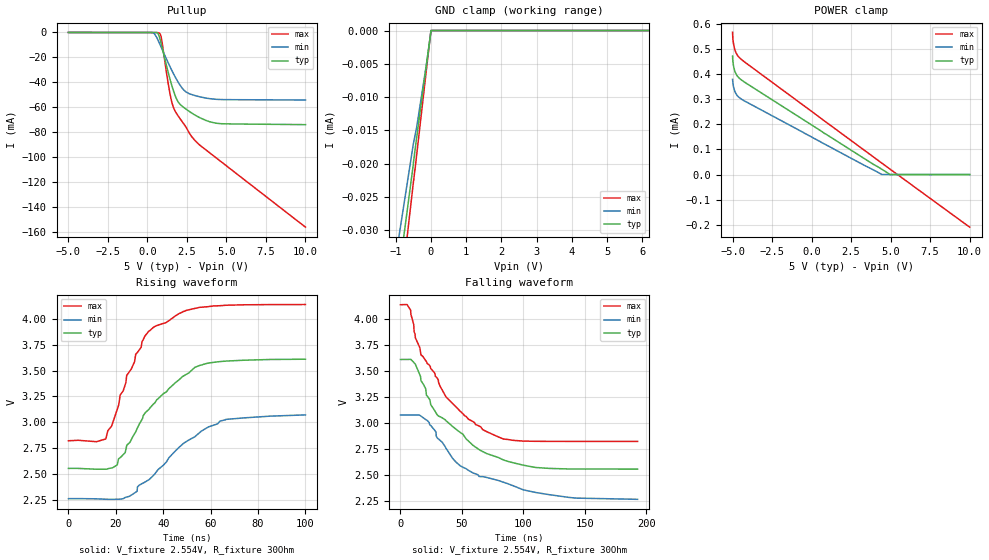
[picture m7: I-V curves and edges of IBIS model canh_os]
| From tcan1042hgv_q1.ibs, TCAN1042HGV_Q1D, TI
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|   canh_os Model
[Model]   canh_os
Model_type   I/O_open_source
Polarity   Inverting
Enable   Active-Low
Vinl = 0.5
Vinh = 0.9
Vmeas = 3
Vref = 2.554
Cref = 2pF
Rref = 30
|   typ   min   max
|   (nom PVT)   (fast PVT)   (slow PVT)
C_comp   8.777e-12   8.206e-12   9.702e-12
| Where nom  PVT is Nominal Process, 5V, 27C
|   Fast PVT is Strong Process,  5.5V, -55C
|   Slow PVT is Weak Process,   4.5V, 150C
[Voltage Range]   5   4.5   5.5
|Junction Temperature
[Temperature Range]   27   150   -55
[Pullup Reference]   5   4.5   5.5
[Pulldown Reference]   0   0   0
[Power Clamp Reference]   5   4.5   5.5
[GND Clamp Reference]   0   0   0
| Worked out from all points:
|   slope of the pullup table from 0 to 0.75 V, typ, clamps not added: 231 ohm
|   falling waveform, V_fixture 2.554V, R_fixture 30Ohm: 20-80 % time 44.1ns typ, 55.6ns min, 39.9ns max; typ from 3.61 V to 2.55 V
|   rising waveform, V_fixture 2.554V, R_fixture 30Ohm: 20-80 % time 21.5ns typ, 23.4ns min, 13.7ns max; typ from 2.55 V to 3.61 V
[GND Clamp]
|   Voltage   I(typ)   I(min)   I(max)
-5V       -202.4uA   -171.2uA   -233.7uA
-3.357V   -134.6uA   -114.5uA   -155.4uA
-500mV    -20.15uA   -17.09uA   -22.94uA
-495.5mV  -19.75uA   -16.97uA   -22.73uA
-455mV    -18.15uA   -15.9uA    -20.94uA
-450.5mV  -17.97uA   -15.78uA   -20.93uA
-405.5mV  -16.14uA   -14.59uA   -18.77uA
-108.5mV  -4.381uA   -4.46uA    -5.008uA
-5mV      -411.1nA   -364.3nA   -280.6nA
-500uV    -238.5nA   0A         0A
45mV      0A         0A         0A
10V       0A         0A         0A
[Pullup]
|   Voltage   I(typ)   I(min)   I(max)
-5V       -31.53uA   57.79uA    -113.1uA
296.5mV   -97.64uA   -126.2uA   -124.8uA
632mV     -357.2uA   -5.205mA   -176.4uA
760mV     -3.756mA   -8.675mA   -653.4uA
875mV     -9.236mA   -11.93mA   -4.145mA
1.354V    -33.92mA   -25.43mA   -43.97mA
1.595V    -44.66mA   -31.72mA   -58.13mA
1.962V    -55.98mA   -40.21mA   -67.2mA
2.295V    -60.05mA   -46.04mA   -73.15mA
2.78V     -64.39mA   -49.67mA   -83.11mA
4.468V    -72.9mA    -53.67mA   -101.6mA
10V       -73.85mA   -54.13mA   -155.9mA
[POWER Clamp]
|   Voltage   I(typ)   I(min)   I(max)
-5V       471uA      378.7uA    565.6uA
-4.984V   454.5uA    368.6uA    544.8uA
-4.95V    436.7uA    352.8uA    525.1uA
-4.901V   421.1uA    339.2uA    508.7uA
-4.819V   405.2uA    325.5uA    490uA
-4.676V   389.9uA    311.9uA    472.8uA
-4.423V   375.4uA    299.2uA    456.6uA
785mV     164.8uA    122.2uA    214.6uA
4.45V     20.79uA    16.54nA    45.11uA
4.97V     0A         0A         21.19uA
10V       0A         0A         -209.3uA
[Ramp]
R_load = 30
|   typ   min   max
dV/dt_r   0.634044/2.15619e-08   0.487958/2.34991e-08   0.790548/1.37727e-08
dV/dt_f   0.634032/4.40581e-08   0.487937/5.56809e-08   0.790542/3.99424e-08
[Falling Waveform]
V_fixture = 2.554V
V_fixture_min = 2.262V
V_fixture_max = 2.821V
R_fixture = 30Ohm
|   Time   V(typ)   V(min)   V(max)
0s        3.611V     3.075V     4.138V
8.277ns   3.612V     3.075V     4.086V
11.99ns   3.567V     3.075V     3.838V
16.63ns   3.412V     3.065V     3.656V
24.63ns   3.176V     2.974V     3.524V
36.93ns   3.022V     2.758V     3.253V
48.77ns   2.906V     2.585V     3.109V
67.01ns   2.722V     2.481V     2.933V
109.9ns   2.57V      2.329V     2.822V
193ns     2.554V     2.262V     2.821V
[Rising Waveform]
V_fixture = 2.554V
V_fixture_min = 2.262V
V_fixture_max = 2.821V
R_fixture = 30Ohm
|   Time   V(typ)   V(min)   V(max)
0s        2.554V     2.262V     2.821V
15.81ns   2.546V     2.256V     2.839V
20.59ns   2.587V     2.256V     3.124V
24.59ns   2.774V     2.277V     3.453V
27.91ns   2.888V     2.316V     3.585V
28.39ns   2.908V     2.324V     3.657V
35.94ns   3.178V     2.487V     3.919V
53.41ns   3.532V     2.862V     4.1V
63.95ns   3.586V     3.012V     4.126V
100ns     3.609V     3.071V     4.138V
